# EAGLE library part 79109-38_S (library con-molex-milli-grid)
RECEPTACAL
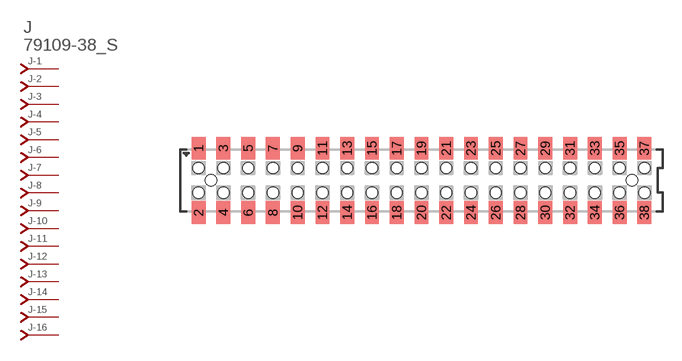
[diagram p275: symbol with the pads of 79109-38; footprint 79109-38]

Designator prefix J; gates -1=J-NV -2=J-N -3=J-N -4=J-N -5=J-N -6=J-N -7=J-N -8=J-N -9=J-N -10=J-N -11=J-N -12=J-N -13=J-N -14=J-N -15=J-N -16=J-N -17=J-N -18=J-N -19=J-N -20=J-N -21=J-N -22=J-N -23=J-N -24=J-N -25=J-N -26=J-N -27=J-N -28=J-N -29=J-N -30=J-N -31=J-N -32=J-N -33=J-N -34=J-N -35=J-N -36=J-N -37=J-N -38=J-N

## 79109-38_S  [79109-38]
1  -1:J  pas
2  -2:J  pas
3  -3:J  pas
4  -4:J  pas
5  -5:J  pas
6  -6:J  pas
7  -7:J  pas
8  -8:J  pas
9  -9:J  pas
10  -10:J  pas
11  -11:J  pas
12  -12:J  pas
13  -13:J  pas
14  -14:J  pas
15  -15:J  pas
16  -16:J  pas
17  -17:J  pas
18  -18:J  pas
19  -19:J  pas
20  -20:J  pas
21  -21:J  pas
22  -22:J  pas
23  -23:J  pas
24  -24:J  pas
25  -25:J  pas
26  -26:J  pas
27  -27:J  pas
28  -28:J  pas
29  -29:J  pas
30  -30:J  pas
31  -31:J  pas
32  -32:J  pas
33  -33:J  pas
34  -34:J  pas
35  -35:J  pas
36  -36:J  pas
37  -37:J  pas
38  -38:J  pas

## Footprint 79109-38 (pad centres in mm)
RECEPTACAL SMD Dual Row, Vertical, Pass-Thru
smd 1.12 x 1.83: 1 -18,2.6; 2 -18,-2.6; 3 -16,2.6; 4 -16,-2.6; 5 -14,2.6; 6 -14,-2.6; 7 -12,2.6; 8 -12,-2.6; 9 -10,2.6; 10 -10,-2.6; 11 -8,2.6; 12 -8,-2.6; 13 -6,2.6; 14 -6,-2.6; 15 -4,2.6; 16 -4,-2.6; 17 -2,2.6; 18 -2,-2.6; 19 0,2.6; 20 0,-2.6; 21 2,2.6; 22 2,-2.6; 23 4,2.6; 24 4,-2.6; 25 6,2.6; 26 6,-2.6; 27 8,2.6; 28 8,-2.6; 29 10,2.6; 30 10,-2.6; 31 12,2.6; 32 12,-2.6; 33 14,2.6; 34 14,-2.6; 35 16,2.6; 36 16,-2.6; 37 18,2.6; 38 18,-2.6
hole 0.914 at -17,0
hole 0.914 at -18,1
hole 0.914 at -18,-1
hole 0.914 at -16,-1
hole 0.914 at -16,1
hole 0.914 at -14,-1
hole 0.914 at -14,1
hole 0.914 at 17,0
hole 0.914 at -12,1
hole 0.914 at -12,-1
hole 0.914 at -10,1
hole 0.914 at -10,-1
hole 0.914 at -8,1
hole 0.914 at -8,-1
hole 0.914 at -6,1
hole 0.914 at -6,-1
hole 0.914 at -4,-1
hole 0.914 at -4,1
hole 0.914 at -2,1
hole 0.914 at -2,-1
hole 0.914 at 0,1
hole 0.914 at 0,-1
hole 0.914 at 2,1
hole 0.914 at 2,-1
hole 0.914 at 4,-1
hole 0.914 at 4,1
hole 0.914 at 6,1
hole 0.914 at 8,1
hole 0.914 at 10,1
hole 0.914 at 6,-1
hole 0.914 at 8,-1
hole 0.914 at 10,-1
hole 0.914 at 12,-1
hole 0.914 at 14,-1
hole 0.914 at 16,-1
hole 0.914 at 18,-1
hole 0.914 at 12,1
hole 0.914 at 14,1
hole 0.914 at 16,1
hole 0.914 at 18,1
